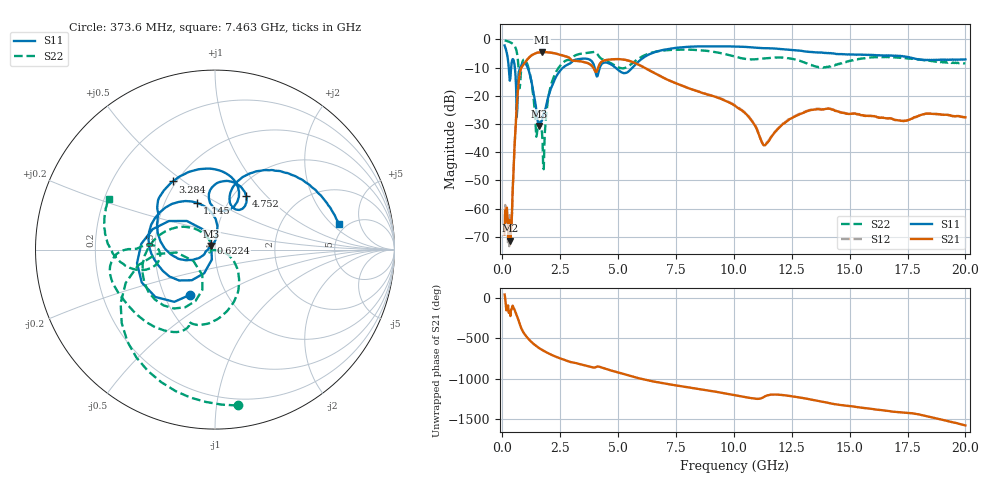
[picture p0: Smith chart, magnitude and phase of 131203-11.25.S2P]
!  2-Port S-parameters saved by WinCal
! VAR MeasName=S-Parameters (CALIBRATED_DATA) read from VNA (N5244A)
! VAR MeasDate=4/4/2013 3:57:50 PM
! VAR NAME=131203-11.25
! VAR FILENAME=131203-11.25.S2P
! VAR DATE=4/4/2013 3:57:50 PM
! VAR PHYS_PORTS=1,2
# Hz S MA R 50
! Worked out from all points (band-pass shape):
!   801 points, 100 MHz to 20 GHz, reference 50 ohm
!   highest |S21| = -4.52 dB at 1.717 GHz (marker M1); lowest = -71.5 dB at 348.8 MHz (marker M2)
!   |S21| within 3 dB of the highest: 1.046 GHz to 3.021 GHz (1.975 GHz wide, 97.1 % of centre); 4.395 GHz to 5.439 GHz (1.044 GHz wide, 21.2 % of centre)
!   lowest |S11| = -30.7 dB at 1.593 GHz (marker M3), VSWR 1.06, Z = 48 + j1.98 ohm
!   |S11| at or under -10 dB: 541.6 MHz to 776.7 MHz (235.1 MHz wide, 35.7 % of centre); 1.096 GHz to 2.628 GHz (1.532 GHz wide, 82.3 % of centre); 4.884 GHz to 5.625 GHz (740.6 MHz wide, 14.1 % of centre)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
!   |S22| runs from -46.1 to -0.4 dB; largest |S21 - S12| = 0.0022
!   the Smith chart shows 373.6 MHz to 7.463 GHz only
!   S11 on the Smith chart (normalised r, x): 373.6 MHz: 0.68, -0.37; 622.4 MHz: 0.96, +0.07; 1.145 GHz: 0.72, +0.41; 3.284 GHz: 0.48, +0.45; 4.752 GHz: 1.13, +0.78; 7.463 GHz: 4.36, +2.42
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1e8  0.7794 -66.7  0.0003473 44.4  0.0003871 -8.3  0.9571 -22.2
3.4875e8  0.2033 -122.7  0.0002675 137.6  0.0005875 -171.4  0.8877 -76.1
3.73625e8  0.287 -118.8  0.0004391 -145.8  0.0005307 -159.3  0.8776 -81.8
6.22375e8  0.04187 119.9  0.06256 149.9  0.06269 150.1  0.6043 -150.5
8.4625e8  0.355 -176.2  0.3271 -30.3  0.3278 -30.2  0.3623 -117.4
1.14475e9  0.2777 110.7  0.4712 -151.6  0.4725 -151.5  0.2969 160.3
1.44325e9  0.0682 84.1  0.5675 130.1  0.5692 130.1  0.02793 132.0
1.5925e9  0.02906 134.9  0.5878 98.7  0.5894 98.6  0.03462 -153.9
1.716875e9  0.03667 176.2  0.5946 76.2  0.5961 76.2  0.02167 -161.1
2.23925e9  0.1831 -161.7  0.5683 0.8  0.5697 0.9  0.2222 -52.8
2.73675e9  0.3416 159.9  0.5002 -53.4  0.5011 -53.5  0.4182 -97.1
3.284e9  0.4467 121.8  0.4133 -95.3  0.4131 -95.3  0.5444 -127.1
3.43325e9  0.4547 111.0  0.4033 -106.4  0.4035 -106.4  0.5595 -135.7
4.751625e9  0.347 60.2  0.4426 176.1  0.4437 176.1  0.3652 175.8
5.5725e9  0.2999 74.3  0.4046 108.8  0.4045 108.8  0.3658 -164.1
6.741625e9  0.6229 38.6  0.232 32.1  0.2315 32.3  0.6166 172.3
7.463e9  0.7042 11.5  0.1684 -3.0  0.1689 -2.6  0.6563 154.5
1.005e10  0.7464 -68.3  0.06637 -127.1  0.06801 -127.0  0.4973 107.6
1.131862e10  0.6966 -101.1  0.01322 -144.7  0.01341 -145.0  0.4594 107.0
1.338325e10  0.5976 -147.9  0.05615 176.2  0.05659 175.1  0.344 85.4
1.669162e10  0.5205 157.7  0.03986 36.9  0.03999 35.3  0.4814 78.6
2e10  0.4425 121.2  0.04136 -142.7  0.04125 -143.8  0.3762 59.3
